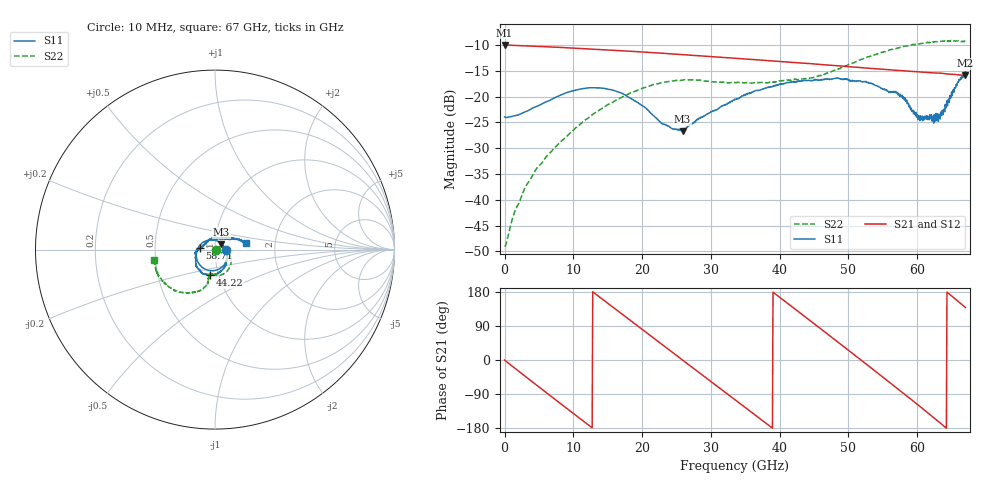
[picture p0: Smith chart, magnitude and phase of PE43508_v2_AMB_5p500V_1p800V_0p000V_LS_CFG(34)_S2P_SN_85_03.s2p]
!Keysight Technologies,N5227A,US51270237,A.10.43.00
!Date: Wednesday, August 22, 2018 17:10:06
!Correction: S11(Full 2 Port(1,3))
!S31(Full 2 Port(1,3))
!S13(Full 2 Port(1,3))
!S33(Full 2 Port(1,3))
!S2P File: Measurements: S11, S31, S13, S33:
# Hz S  dB  R 50
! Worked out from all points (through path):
!   801 points, 10 MHz to 67 GHz, reference 50 ohm
!   highest |S21| = -9.95 dB at 10 MHz (marker M1); lowest = -15.9 dB at 67 GHz (marker M2)
!   group delay of S21, straight-line fit = 38.7 ps
!   lowest |S11| = -26.7 dB at 25.88 GHz (marker M3), VSWR 1.10, Z = 53.5 + j3.28 ohm
!   |S11| at or under -10 dB: start of sweep to end of sweep
!   |S22| runs from -49.0 to -9.1 dB; largest |S21 - S12| = 0.0017
!   S11 on the Smith chart (normalised r, x): 10 MHz: 1.14, -0.00; 44.22 GHz: 0.91, -0.26; 58.71 GHz: 0.84, +0.01; 67 GHz: 1.41, +0.11
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1e7  -23.93 -0.7  -9.95 -0.2  -9.95 -0.2  -48.96 -3.0
1.601012e9  -23.67 -9.7  -10.06 -23.2  -10.05 -23.2  -41.86 43.1
4.448088e9  -21.98 -30.0  -10.22 -63.4  -10.22 -63.4  -34.36 40.1
7.630112e9  -20.01 -60.1  -10.41 -108.0  -10.41 -107.9  -29.44 29.0
1.123082e10  -18.47 -98.2  -10.65 -158.0  -10.65 -158.0  -25.08 7.7
1.416164e10  -18.34 -131.0  -10.86 161.4  -10.86 161.4  -22.28 -9.1
1.74274e10  -19.59 -169.9  -11.11 116.3  -11.11 116.3  -19.85 -28.3
1.985579e10  -21.58 156.7  -11.31 82.7  -11.30 82.7  -18.44 -42.3
2.236791e10  -24.57 116.3  -11.53 48.1  -11.52 48.1  -17.44 -57.2
2.588489e10  -26.67 41.3  -11.85 -0.3  -11.84 -0.3  -16.77 -75.9
2.998802e10  -22.92 -20.4  -12.23 -56.6  -12.23 -56.6  -17.04 -91.0
3.3505e10  -20.58 -48.2  -12.55 -104.9  -12.55 -104.9  -17.27 -98.0
3.878046e10  -18.07 -75.9  -13.03 -177.6  -13.04 -177.5  -17.08 -101.2
4.42234e10  -16.83 -100.4  -13.58 106.8  -13.57 106.8  -16.42 -102.8
4.472582e10  -16.87 -102.7  -13.61 99.7  -13.60 99.8  -16.33 -102.7
4.748916e10  -16.65 -114.2  -13.91 61.1  -13.91 61.0  -15.18 -102.2
5.067119e10  -16.97 -128.0  -14.24 16.2  -14.23 16.3  -13.46 -104.6
5.586291e10  -19.19 -161.8  -14.75 -57.5  -14.75 -57.8  -10.98 -121.1
5.870999e10  -21.26 174.6  -15.06 -98.3  -15.07 -98.4  -10.15 -132.0
6.046848e10  -23.71 142.2  -15.21 -123.8  -15.22 -124.0  -9.70 -139.3
6.29806e10  -23.31 80.4  -15.41 -160.7  -15.42 -161.1  -9.35 -151.0
6.7e10  -15.14 12.3  -15.88 138.5  -15.95 138.5  -9.26 -170.0
